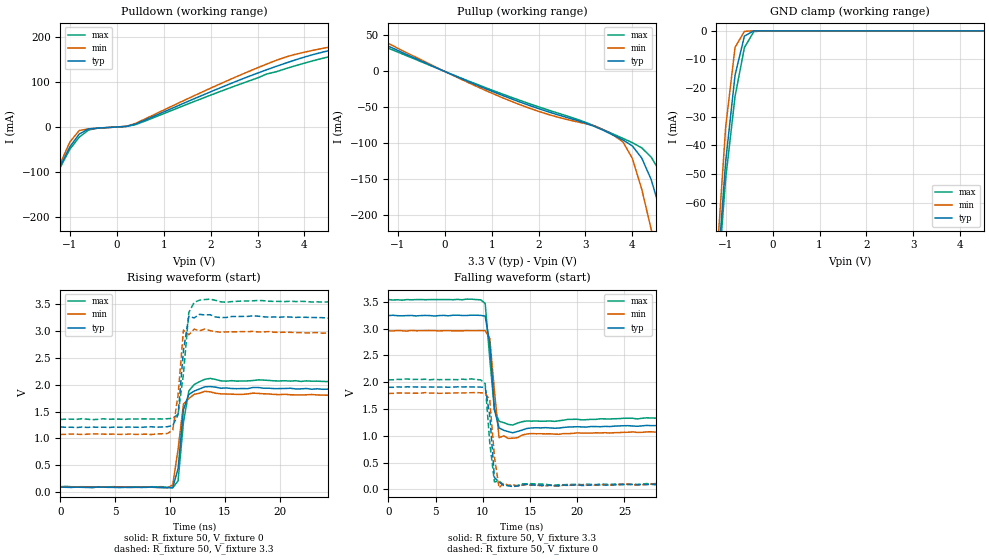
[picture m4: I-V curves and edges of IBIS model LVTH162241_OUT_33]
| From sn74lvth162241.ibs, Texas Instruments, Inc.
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|  Model LVTH162241 Output_33
[Model]   LVTH162241_OUT_33
Model_type  3-state
Polarity   Non-Inverting
Enable   Active-Low
Vmeas = 1.5V
Cref = 50pF
Rref = 500
Vref = 0
| variable   typ   min   max
C_comp   9pf   NA   NA
[Temperature Range]   40   -25   100
| Ambient temperature   25   -40   85
[Voltage range]   3.3   3.0   3.6
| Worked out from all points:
|   slope of the pulldown table from 0 to 0.495 V, typ, clamps not added: 46.2 ohm
|   slope of the pullup table from 0 to 0.495 V, typ, clamps not added: 35.8 ohm
|   GND clamp passes 1 mA (typ) near -0.51 V on its own axis
|   rising waveform, R_fixture 50, V_fixture 0: 20-80 % time 486ps typ, 651ps min, 668ps max; typ from 0.091 V to 1.9 V
|   falling waveform, R_fixture 50, V_fixture 3.3: 20-80 % time 550ps typ, 589ps min, 650ps max; typ from 3.24 V to 1.21 V
|   rising waveform, R_fixture 50, V_fixture 3.3: 20-80 % time 567ps typ, 578ps min, 653ps max; typ from 1.21 V to 3.24 V
|   falling waveform, R_fixture 50, V_fixture 0: 20-80 % time 547ps typ, 541ps min, 602ps max; typ from 1.91 V to 0.092 V
[Pullup]
|  Voltage   I(typ)   I(min)   I(max)
-5V       94.23uA    85.85uA    99.01uA
-2V       82.01uA    71.47uA    88.83uA
-1.8V     81.6uA     58.6mA     88.39uA
-1.6V     81.15uA    52.4mA     87.97uA
-1.4V     40.89mA    45.94mA    37.61mA
1.2V      -32.56mA   -35.68mA   -30.64mA
3.6V      -88.69mA   -88.73mA   -87.23mA
4V        -103.5mA   -120.9mA   -98.99mA
4.4V      -150mA     -219mA     -119mA
4.6V      -194.6mA   -274.3mA   -140.7mA
5V        -293.7mA   -384.9mA   -221mA
10V       -1.532A    -1.768A    -1.403A
[Pulldown]
|   Voltage   I(typ)   I(min)   I(max)
-5V       -1.45A     -1.689A    -1.258A
-1.8V     -293.1mA   -319.2mA   -269.1mA
-1.6V     -220.8mA   -233.6mA   -207.3mA
-1.2V     -86.47mA   -80.77mA   -89.3mA
-1V       -44.25mA   -33.52mA   -49.79mA
-800mV    -15.95mA   -7.942mA   -22.7mA
-600mV    -4.327mA   -4.262mA   -6.948mA
400mV     6.383mA    7.977mA    5.131mA
3.6V      142mA      155.5mA    129.6mA
5.2V      182.7mA    189.8mA    170.3mA
7.2V      209.9mA    220.9mA    195.1mA
10V       244.6mA    264mA      221.4mA
[GND Clamp]
|   Voltage   I(typ)   I(min)   I(max)
-5V       -1.539A    -1.735A    -1.331A
-1.2V     -90.42mA   -82.39mA   -94.21mA
-1V       -45.59mA   -33.58mA   -51.59mA
-800mV    -15.44mA   -5.752mA   -22.87mA
-600mV    -1.841mA   -182.4uA   -5.815mA
-400mV    -8.289uA   -83.28nA   -283.7uA
-200mV    -5.336nA   -26.79nA   -824.4nA
5V        42.74nA    481.9nA    79.44nA
[Ramp]
| variable   typ   min   max
dV/dt_r   1.116E+00/4.680E-10  1.050E+00/4.550E-10  1.200E+00/4.910E-10
dV/dt_f   1.254E+00/4.990E-10  1.158E+00/4.260E-10  1.344E+00/5.360E-10
R_load = 50
[Rising Waveform]
R_fixture = 50
V_fixture = 0
V_fixture_min = 0
V_fixture_max = 0
C_fixture = 0
L_fixture = 0
|   Time   V(typ)   V(min)   V(max)
0s        90.94mV    88.65mV    97.66mV
9.766ns   83.16mV    77.36mV    85.15mV
10.25ns   79.5mV     131.7mV    76.91mV
10.74ns   435mV      796.8mV    207.8mV
11.23ns   1.536V     1.64V      1.3V
11.72ns   1.818V     1.742V     1.883V
12.21ns   1.882V     1.821V     2.004V
13.18ns   1.961V     1.877V     2.101V
30.76ns   1.904V     1.78V      2.044V
49.71ns   1.9V       1.793V     2.053V
[Falling Waveform]
R_fixture = 50
V_fixture = 3.3
V_fixture_min = 3.0
V_fixture_max = 3.6
C_fixture = 0
L_fixture = 0
|   Time   V(typ)   V(min)   V(max)
0s        3.242V     2.957V     3.539V
8.789ns   3.249V     2.959V     3.547V
10.25ns   3.232V     2.96V      3.468V
10.74ns   2.719V     2.814V     2.434V
11.23ns   1.486V     1.837V     1.489V
11.72ns   1.147V     965.4mV    1.272V
12.7ns    1.078V     951.4mV    1.213V
15.14ns   1.146V     1.042V     1.273V
32.23ns   1.205V     1.088V     1.36V
49.71ns   1.21V      1.077V     1.353V
[Rising Waveform]
R_fixture = 50
V_fixture = 3.3
V_fixture_min = 3.0
V_fixture_max = 3.6
C_fixture = 0
L_fixture = 0
|   Time   V(typ)   V(min)   V(max)
0s        1.212V     1.074V     1.353V
9.766ns   1.217V     1.091V     1.366V
10.25ns   1.238V     1.154V     1.375V
10.74ns   1.441V     1.803V     1.449V
11.23ns   2.639V     3.019V     2.205V
11.72ns   3.274V     2.931V     3.348V
12.21ns   3.246V     3.036V     3.535V
12.7ns    3.313V     3.005V     3.577V
14.65ns   3.252V     2.979V     3.545V
49.71ns   3.238V     2.952V     3.537V
[Falling Waveform]
R_fixture = 50
V_fixture = 0
V_fixture_min = 0
V_fixture_max = 0
C_fixture = 0
L_fixture = 0
|   Time   V(typ)   V(min)   V(max)
0s        1.905V     1.79V      2.043V
8.789ns   1.911V     1.803V     2.062V
9.766ns   1.908V     1.802V     2.042V
10.25ns   1.902V     1.797V     1.975V
10.74ns   1.376V     1.662V     862.4mV
11.23ns   222.9mV    608.5mV    140.1mV
11.72ns   137mV      29.45mV    159.2mV
12.21ns   74.92mV    117.8mV    84.38mV
13.67ns   64.85mV    60.12mV    75.38mV
49.71ns   92.32mV    91.71mV    101.9mV
